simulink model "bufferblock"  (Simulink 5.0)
settings: Solver=ode45  StartTime=0.0  StopTime=8  RelTol=1e-3

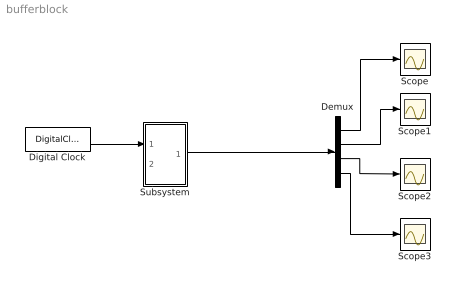
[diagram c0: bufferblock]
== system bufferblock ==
  Demux : Demux
  Digital Clock : DigitalClock
  Scope{,1..3} (4 alike) : Scope
  Subsystem : Subsystem
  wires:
  Subsystem/1(Out1) -> Demux/1
  Demux/1 -> Scope/1
  Demux/2 -> Scope1/1
  Demux/3 -> Scope2/1
  Demux/4 -> Scope3/1
  Digital Clock/1 -> Subsystem/1(In1)

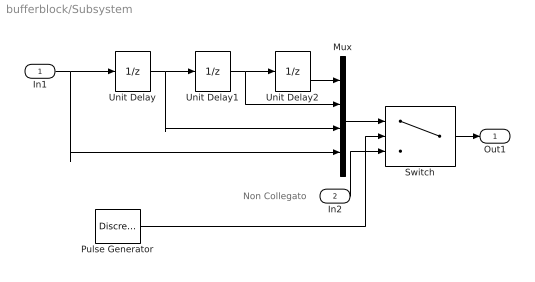
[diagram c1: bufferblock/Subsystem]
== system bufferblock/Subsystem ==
  note: Non Collegato
  In1 : Inport
  In2 : Inport  Port=2
  Mux : Mux
  Pulse Generator : DiscretePulseGenerator  PulseType=Time based  Period=4  PulseWidth=0.1
  Switch : Switch  Threshold=1
  Unit Delay : UnitDelay
  Unit Delay1 : UnitDelay
  Unit Delay2 : UnitDelay
  Out1 : Outport
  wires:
  Unit Delay/1 -> Unit Delay1/1, Mux/3
  Unit Delay1/1 -> Unit Delay2/1, Mux/2
  In1/1 -> Mux/4, Unit Delay/1
  Unit Delay2/1 -> Mux/1
  Mux/1 -> Switch/1
  Pulse Generator/1 -> Switch/2
  Switch/1 -> Out1/1
  In2/1 -> Switch/3
